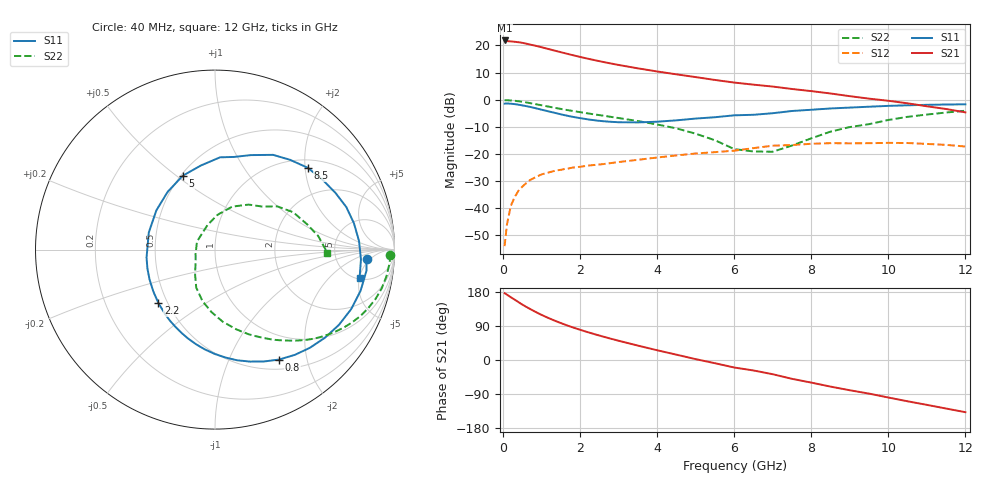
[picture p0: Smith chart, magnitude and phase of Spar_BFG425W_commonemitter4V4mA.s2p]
! Filename: 44bfg425.001
! BFG425W Field C1
! V1=8.166E-001V,V2=4.000E+000V, I1=3.940E-005A, I2=4.000E-003A
# GHz  S  MA  R 50
!  S11  S21  S12  S22
!Freq(GHz)  Mag  Ang  Mag  Ang  Mag  Ang  Mag  Ang
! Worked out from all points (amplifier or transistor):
!   44 points, 40 MHz to 12 GHz, reference 50 ohm
!   highest |S21| = 21.8 dB at 40 MHz (marker M1)
!   |S21| within 3 dB of that: start of sweep to 1.136 GHz
!   unconditionally stable (mu >= 1): 2.621 GHz to end of sweep
!   at 700 MHz: K = 0.31, MSG = 25.0 dB, |S12| = -29.6 dB
!   at 2.4 GHz: K = 0.92, MSG = 19.3 dB, |S12| = -24.0 dB
!   at 12 GHz: K = 1.56, MAG = 1.9 dB, |S12| = -17.3 dB
!   S11 on the Smith chart (normalised r, x): 40 MHz: 11, -4; 800 MHz: 0.63, -1.55; 2.2 GHz: 0.45, -0.33; 5 GHz: 0.51, +0.53; 8.5 GHz: 1.19, +2.06; 12 GHz: 5.20, -5.04
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0.04  0.846 -3.4  12.34 176.2  0.002 50.3  0.977 -1.6
0.2  0.843 -15.8  11.86 165.7  0.011 74.8  0.967 -8.8
0.3  0.828 -23.6  11.67 159.4  0.016 72.0  0.954 -13.0
0.5  0.785 -38.7  11.16 146.2  0.025 64.7  0.914 -20.9
0.6  0.761 -45.9  10.77 140.3  0.029 61.2  0.891 -24.5
0.8  0.709 -59.8  10.01 129.2  0.036 54.4  0.839 -31.2
1.1  0.629 -78.7  8.867 114.3  0.044 46.2  0.764 -39.6
1.3  0.581 -90.2  8.146 105.5  0.048 41.9  0.718 -44.4
1.5  0.538 -101.3  7.495 97.4  0.051 38.3  0.676 -48.6
1.8  0.484 -117.0  6.631 86.4  0.056 34.1  0.621 -54.4
2.2  0.434 -136.6  5.693 73.4  0.061 29.7  0.559 -61.6
2.6  0.401 -155.3  4.952 61.7  0.065 26.4  0.507 -68.4
3  0.384 -173.3  4.363 50.8  0.071 23.4  0.459 -75.1
3.5  0.381 165.5  3.778 38.0  0.078 19.5  0.404 -83.9
4.5  0.416 129.4  2.931 14.0  0.094 10.2  0.296 -103.5
5  0.449 113.6  2.607 2.3  0.102 3.6  0.236 -116.3
6  0.515 86.9  2.067 -19.8  0.115 -9.3  0.123 -151.2
6.5  0.527 78.4  1.892 -27.6  0.128 -9.7  0.111 -167.1
7.5  0.619 58.5  1.574 -49.7  0.146 -28.4  0.143 107.1
8.5  0.689 41.5  1.301 -70.2  0.158 -45.2  0.258 68.2
10.5  0.788 10.7  0.857 -109.0  0.159 -80.6  0.483 25.5
12  0.821 -11.1  0.584 -137.7  0.137 -112.1  0.626 -1.6
